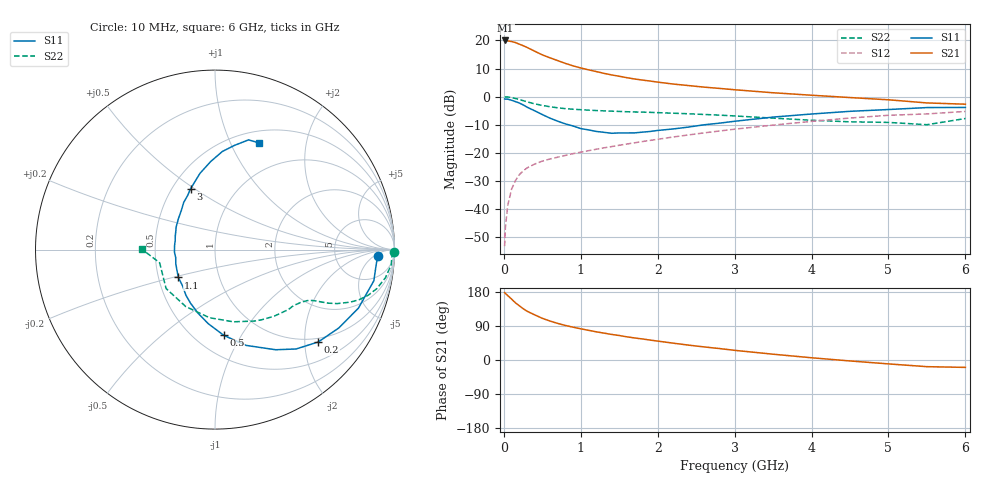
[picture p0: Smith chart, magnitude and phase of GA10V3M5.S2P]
! Infineon Technologies  Discrete & RF Semiconductors
! BF775
! Si NPN RF Bipolar Junction Transistor in SOT23
! VCE = 10 V  IC = 3.5 mA
! Common Emitter S-Parameters:  May  1996
# GHz  S  MA  R  50
!  f  S11  S21  S12  S22
! GHz  MAG  ANG  MAG  ANG  MAG  ANG  MAG  ANG
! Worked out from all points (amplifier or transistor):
!   36 points, 10 MHz to 6 GHz, reference 50 ohm
!   highest |S21| = 20.0 dB at 20 MHz (marker M1)
!   |S21| within 3 dB of that: start of sweep to 340.1 MHz
!   unconditionally stable (mu >= 1): 991.7 MHz to 3.077 GHz
!   at 250 MHz: K = 0.37, MSG = 22.3 dB, |S12| = -26.4 dB
!   at 1.4 GHz: K = 1.10, MAG = 10.8 dB, |S12| = -17.8 dB
!   at 6 GHz: K = 0.89, MSG = 1.3 dB, |S12| = -5.3 dB
!   S11 on the Smith chart (normalised r, x): 10 MHz: 18, -7; 200 MHz: 0.91, -2.31; 500 MHz: 0.68, -0.84; 1.1 GHz: 0.63, -0.21; 3 GHz: 0.62, +0.48; 6 GHz: 0.64, +1.29
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0.01  0.9101 -2.1  9.899 177.9  0.0022 86.7  0.9968 -0.9
0.02  0.9027 -4.6  9.966 175.6  0.0047 85.3  0.9867 -1.9
0.05  0.9019 -11.1  9.789 170.1  0.0115 82.3  0.9854 -4.9
0.1  0.8631 -22.2  9.534 160.9  0.0226 77.7  0.9624 -9.4
0.15  0.8165 -32.3  9.148 151.0  0.032 72.1  0.927 -13.6
0.2  0.7719 -41.8  8.582 143.3  0.0408 68.1  0.8902 -16.6
0.25  0.7146 -50.8  8.064 135.6  0.0477 63.9  0.8497 -19.2
0.3  0.6523 -58.8  7.508 129.0  0.0539 61.3  0.8091 -21.2
0.4  0.5612 -72.0  6.429 119.2  0.0633 57.5  0.7453 -23.8
0.5  0.4805 -84.1  5.527 110.0  0.0715 55.5  0.6983 -25.3
0.6  0.4144 -95.2  4.9 102.8  0.078 54.4  0.6613 -26.2
0.7  0.3662 -105.1  4.367 96.6  0.0839 54.5  0.6332 -26.9
0.8  0.3277 -114.7  3.899 91.2  0.0902 54.2  0.6122 -27.6
1.1  0.2567 -142.8  2.996 78.4  0.1094 55.1  0.5756 -30.1
1.3  0.2323 -160.1  2.596 71.0  0.1231 55.8  0.5589 -31.9
1.6  0.2264 174.3  2.171 61.1  0.1439 56.4  0.5391 -35.3
2.2  0.2665 140.0  1.675 44.5  0.1917 55.5  0.5076 -44.5
3  0.3651 111.9  1.326 25.5  0.264 50.9  0.4539 -61.3
3.5  0.4333 101.1  1.172 15.3  0.312 46.4  0.415 -75.8
4.5  0.5483 85.7  0.963 -2.5  0.4168 35.0  0.3567 -117.1
5.5  0.6394 73.0  0.773 -17.6  0.4929 19.3  0.3171 -166.6
6  0.6429 67.6  0.734 -19.5  0.546 14.9  0.4085 179.5
